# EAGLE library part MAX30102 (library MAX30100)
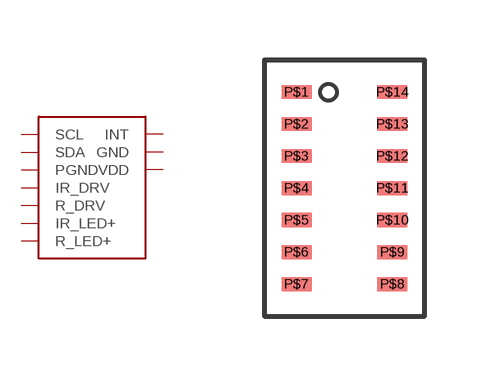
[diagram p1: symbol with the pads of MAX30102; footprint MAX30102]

Designator prefix -

## MAX30102  [MAX30102]
P$2  SCL
P$3  SDA
P$4  PGND
P$5  R_DRV
P$6  IR_DRV
P$9  R_LED+
P$10  IR_LED+
P$11  VDD
P$12  GND
P$13  INT

## Footprint MAX30102 (pad centres in mm)
smd 0.75 x 0.35: P$1 0,4.8; P$2 0,4; P$3 0,3.2; P$4 0,2.4; P$5 0,1.6; P$6 0,0.8; P$7 0,0; P$8 2.4,0; P$9 2.4,0.8; P$10 2.4,1.6; P$11 2.4,2.4; P$12 2.4,3.2; P$13 2.4,4; P$14 2.4,4.8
